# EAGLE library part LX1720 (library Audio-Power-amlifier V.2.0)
The LX1720 is a highly-integrated, Switching Class-D Stereo Power Amplifier Controller IC with power and size features that make it ideal for multimedia computer applications, as well as other applications where high fidelity sound is required. With input voltage ranging from 7V- 15V, the LX1720 is designed to operate over the full 20Hz to 20kHz audio range. Signal distortion measurements using industry standard 1kHz signal yields THD + noise levels < 1% (10 watts output).
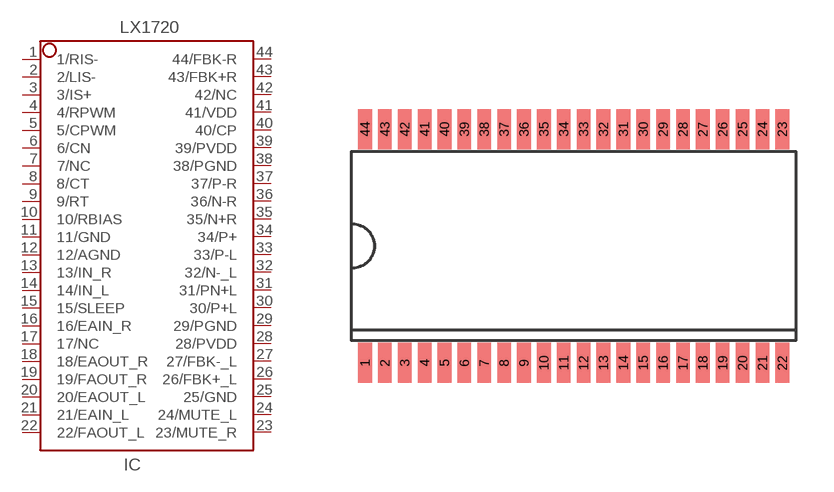
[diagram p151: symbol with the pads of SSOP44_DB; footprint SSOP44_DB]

Designator prefix IC

## LX1720  [SSOP44_DB]
1  1/RIS-  in
2  2/LIS-  in
3  3/IS+  in
4  4/RPWM
5  5/CPWM
6  6/CN  out
7  7/NC  nc
8  8/CT
9  9/RT
10  10/RBIAS
11  11/GND  pwr
12  12/AGND  pwr
13  13/IN_R  in
14  14/IN_L  in
15  15/SLEEP  in
16  16/EAIN_R  in
17  17/NC  nc
18  18/EAOUT_R  out
19  19/FAOUT_R  out
20  20/EAOUT_L  out
21  21/EAIN_L  in
22  22/FAOUT_L  out
23  23/MUTE_R  in
24  24/MUTE_L  in
25  25/GND  pwr
26  26/FBK+_L  in
27  27/FBK-_L  in
28  28/PVDD  out
29  29/PGND  pwr
30  30/P+L  out
31  31/PN+L  out
32  32/N-_L  out
33  33/P-L  out
34  34/P+  out
35  35/N+R  out
36  36/N-R  out
37  37/P-R  out
38  38/PGND  pwr
39  39/PVDD  out
40  40/CP  out
41  41/VDD  pwr
42  42/NC  pwr
43  43/FBK+R  in
44  44/FBK-R  in

## Footprint SSOP44_DB (pad centres in mm)
SSOP044_DB_7,5X17,83X0,8
smd 0.55 x 1.6: 1 -8.4,-4.7; 2 -7.6,-4.7; 3 -6.8,-4.7; 4 -6,-4.7; 5 -5.2,-4.7; 6 -4.4,-4.7; 7 -3.6,-4.7; 8 -2.8,-4.7; 9 -2,-4.7; 10 -1.2,-4.7; 11 -0.4,-4.7; 12 0.4,-4.7; 13 1.2,-4.7; 14 2,-4.7; 15 2.8,-4.7; 16 3.6,-4.7; 17 4.4,-4.7; 18 5.2,-4.7; 19 6,-4.7; 20 6.8,-4.7; 21 7.6,-4.7; 22 8.4,-4.7; 23 8.4,4.7; 24 7.6,4.7; 25 6.8,4.7; 26 6,4.7; 27 5.2,4.7; 28 4.4,4.7; 29 3.6,4.7; 30 2.8,4.7; 31 2,4.7; 32 1.2,4.7; 33 0.4,4.7; 34 -0.4,4.7; 35 -1.2,4.7; 36 -2,4.7; 37 -2.8,4.7; 38 -3.6,4.7; 39 -4.4,4.7; 40 -5.2,4.7; 41 -6,4.7; 42 -6.8,4.7; 43 -7.6,4.7; 44 -8.4,4.7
